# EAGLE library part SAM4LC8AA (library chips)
Atmel SAM4L microcontroller. ARM Cortex M4 with 512 KB Flash and 64 KB RAM
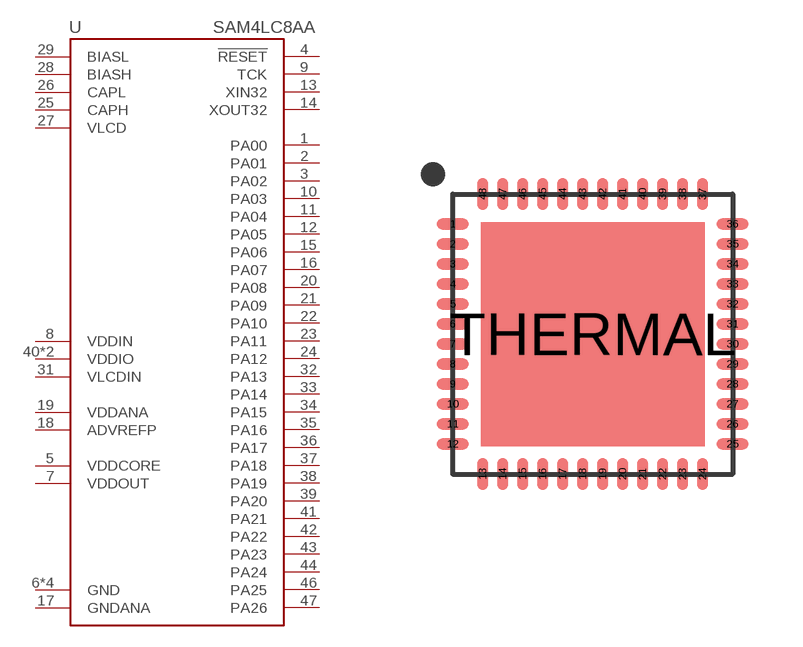
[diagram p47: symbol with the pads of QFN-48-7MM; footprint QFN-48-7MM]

Designator prefix U

## SAM4LC8AA (DIGIKEY: ATSAM4LC8AA-MU-ND; MANUFACTURER: Microchip Technology; MPN: ATSAM4LC8AA-MU)  [QFN-48-7MM]
1  PA00
2  PA01
3  PA02
4  !RESET
5  VDDCORE  pwr
6  GND  pwr
7  VDDOUT  pwr
8  VDDIN  pwr
9  TCK
10  PA03
11  PA04
12  PA05
13  XIN32
14  XOUT32
15  PA06
16  PA07
17  GNDANA  pwr
18  ADVREFP
19  VDDANA  pwr
20  PA08
21  PA09
22  PA10
23  PA11
24  PA12
25  CAPH
26  CAPL
27  VLCD
28  BIASH
29  BIASL
30  GND  pwr
31  VLCDIN  pwr
32  PA13
33  PA14
34  PA15
35  PA16
36  PA17
37  PA18
38  PA19
39  PA20
40  VDDIO  pwr
41  PA21
42  PA22
43  PA23
44  PA24
45  VDDIO  pwr
46  PA25
47  PA26
48  GND  pwr
THERMAL  GND  pwr

## Footprint QFN-48-7MM (pad centres in mm)
7MM x 7MM 48 QFN package
smd 0.8 x 0.28: 1 -3.5,2.75; 2 -3.5,2.25; 3 -3.5,1.75; 4 -3.5,1.25; 5 -3.5,0.75; 6 -3.5,0.25; 7 -3.5,-0.25; 8 -3.5,-0.75; 9 -3.5,-1.25; 10 -3.5,-1.75; 11 -3.5,-2.25; 12 -3.5,-2.75; 25 3.5,-2.75; 26 3.5,-2.25; 27 3.5,-1.75; 28 3.5,-1.25; 29 3.5,-0.75; 30 3.5,-0.25; 31 3.5,0.25; 32 3.5,0.75; 33 3.5,1.25; 34 3.5,1.75; 35 3.5,2.25; 36 3.5,2.75
smd 0.28 x 0.8: 13 -2.75,-3.5; 14 -2.25,-3.5; 15 -1.75,-3.5; 16 -1.25,-3.5; 17 -0.75,-3.5; 18 -0.25,-3.5; 19 0.25,-3.5; 20 0.75,-3.5; 21 1.25,-3.5; 22 1.75,-3.5; 23 2.25,-3.5; 24 2.75,-3.5; 37 2.75,3.5; 38 2.25,3.5; 39 1.75,3.5; 40 1.25,3.5; 41 0.75,3.5; 42 0.25,3.5; 43 -0.25,3.5; 44 -0.75,3.5; 45 -1.25,3.5; 46 -1.75,3.5; 47 -2.25,3.5; 48 -2.75,3.5
smd 5.6 x 5.6: THERMAL 0,0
